(* Logix 5000 DataType export Banner_ISD_Remote_Block_Data_v1; software revision 36.00 *)

TYPE Banner_Chain_Status_v1 :
STRUCT
   Device_Count_Mismatch : BOOL;   // 0 = False, 1 = True
   Device_Order_Mismatch : BOOL;   // 0 = False, 1 = True
   No_Diagnostics_Data_Detected : BOOL;   // 0 = False, 1 = True
   bit3 : BOOL;
   Incompatible_Device : BOOL;   // 0 = False, 1 = True
   ISD_Terminator_Missing : BOOL;   // 0 = False, 1 = True
   ISD_Actuator_Not_Taught : BOOL;   // 0 = False, 1 = True
   ISD_Wrong_Actuator : BOOL;   // 0 = False, 1 = True
   ISD_Internal_Error : BOOL;   // 0 = False, 1 = True
   ISD_Output_Fault_Detected : BOOL;   // 0 = False, 1 = True
   ISD_Chain_Change_Detected : BOOL;   // 0 = False, 1 = True
   bit11 : BOOL;
   ISD_OSSD_Status : BOOL;   // 0 = Off, 1 = ON
   bit13 : BOOL;
   bit14 : BOOL;
   bit15 : BOOL;
   bit16 : BOOL;
   bit17 : BOOL;
   bit18 : BOOL;
   bit19 : BOOL;
   bit20 : BOOL;
   bit21 : BOOL;
   bit22 : BOOL;
   bit23 : BOOL;
   bit24 : BOOL;
   bit25 : BOOL;
   bit26 : BOOL;
   bit27 : BOOL;
   bit28 : BOOL;
   bit29 : BOOL;
   bit30 : BOOL;
   bit31 : BOOL;
END_STRUCT
END_TYPE

TYPE Banner_ISD_Chains_v1 :
STRUCT
   C1 : DINT;
   C2 : DINT;
   C3 : DINT;
   C4 : DINT;
   C5 : DINT;
   C6 : DINT;
END_STRUCT
END_TYPE

TYPE Banner_ISD_Remote_Block_Data_v1 :
STRUCT
   Device_Count : Banner_ISD_Chains_v1;
   On_Off : Banner_ISD_Chains_v1;
   Fault : Banner_ISD_Chains_v1;
   Marginal : Banner_ISD_Chains_v1;
   Alert : Banner_ISD_Chains_v1;
   Reset : Banner_ISD_Chains_v1;
   Recognized : Banner_ISD_Chains_v1;
   Guard_Lock_Status : Banner_ISD_Chains_v1;
   Status : Banner_ISD_Status_v1;
END_STRUCT
END_TYPE

TYPE Banner_ISD_Status_v1 :
STRUCT
   C1_Status : Banner_Chain_Status_v1;
   C2_Status : Banner_Chain_Status_v1;
   C3_Status : Banner_Chain_Status_v1;
   C4_Status : Banner_Chain_Status_v1;
   C5_Status : Banner_Chain_Status_v1;
   C6_Status : Banner_Chain_Status_v1;
END_STRUCT
END_TYPE
